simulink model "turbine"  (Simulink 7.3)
settings: Solver=ode23tb  StartTime=0.0  StopTime=1000  RelTol=1e-3
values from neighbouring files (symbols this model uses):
  c_d = 0.9658    [dynamic_main.m]    (also in Parameter.m = 1; Parameter_sim.m; static_main.m = inv(H3'*H3)*H3'*y3)
  d_Turb = 5.35    [dynamic_main.m]    (also in Parameter.m; Parameter_sim.m; static_main.m)
  I_IC = 0    [dynamic_main.m]    (also in Parameter.m; Parameter_sim.m; static_main.m)
  kappa = 8.7000e3    (= 8700)    [dynamic_main.m]    (also in Parameter.m = 1; Parameter_sim.m; static_main.m = inv(H4'*H4)*H4'*y4)
  L_net = 0.1    [dynamic_main.m]    (also in Parameter_sim.m; static_main.m)
  L_tot = L_net+L_G    (= 0.2)    [dynamic_main.m]    (also in Parameter.m; Parameter_sim.m)
  omega_IC = 0    [dynamic_main.m]    (also in Parameter.m; Parameter_sim.m; static_main.m)
  p_0 = 0    [dynamic_main.m]    (also in Parameter.m; Parameter_sim.m; static_main.m)
  R_net = 165    [dynamic_main.m]    (also in Parameter_sim.m; static_main.m)
  R_tot = R_net+R_G    (= 175)    [dynamic_main.m]    (also in Parameter.m; Parameter_sim.m)
  rho = 1000    [dynamic_main.m]    (also in Parameter.m; Parameter_sim.m; static_main.m)
  Theta = fminsearch(@(Theta)err_turbine(Theta,time_bb,p_F_bb,x_bb,omega_bb),Theta_0)    [dynamic_main.m]    (also in Parameter.m = 1; Parameter_sim.m = 5499.7)

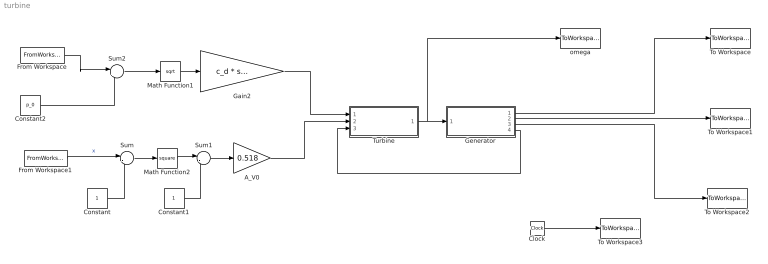
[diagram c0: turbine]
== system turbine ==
  A_V0 : Gain  Gain=0.518  ParameterDataType=sfix(16)  ParameterScaling=2^0  OutDataType=sfix(16)  OutScaling=2^0
  Clock : Clock
  Constant : Constant  OutDataType=sfix(16)  OutScaling=2^0
  Constant1 : Constant  OutDataType=sfix(16)  OutScaling=2^0
  Constant2 : Constant  Value=p_0  OutDataType=sfix(16)  OutScaling=2^0
  From Workspace : FromWorkspace  VariableName=[time_bb p_F_bb]  SampleTime=0
  From Workspace1 : FromWorkspace  VariableName=[time_bb x_bb]  SampleTime=0
  Gain2 : Gain  Gain=c_d * sqrt(2/rho)  ParameterDataType=sfix(16)  ParameterScaling=2^0  OutDataType=sfix(16)  OutScaling=2^0
  Generator : Subsystem
  Math Function1 : Math  Operator=sqrt  OutDataType=sfix(16)  OutScaling=2^0
  Math Function2 : Math  Operator=square  OutDataType=sfix(16)  OutScaling=2^0
  Sum : Sum  Inputs=|-+  OutDataType=sfix(16)  OutScaling=2^0
  Sum1 : Sum  Inputs=|-+  OutDataType=sfix(16)  OutScaling=2^0
  Sum2 : Sum  Inputs=|+-  OutDataType=sfix(16)  OutScaling=2^0
  To Workspace : ToWorkspace  VariableName=U  SampleTime=-1  SaveFormat=Array
  To Workspace1 : ToWorkspace  VariableName=I  SampleTime=-1  SaveFormat=Array
  To Workspace2 : ToWorkspace  VariableName=P  SampleTime=-1  SaveFormat=Array
  To Workspace3 : ToWorkspace  VariableName=time_sim  SampleTime=-1  SaveFormat=Array
  Turbine : Subsystem
  omega : ToWorkspace  VariableName=omega  SampleTime=-1  SaveFormat=Array
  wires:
  Turbine/1(omega) -> Generator/1(omega), omega/1
  Generator/1(U) -> To Workspace/1
  Generator/2(I) -> To Workspace1/1
  Generator/4(T_G) -> Turbine/3(T_G)
  Generator/3(P) -> To Workspace2/1
  Clock/1 -> To Workspace3/1
  Constant2/1 -> Sum2/2
  Sum2/1 -> Math Function1/1
  Math Function1/1 -> Gain2/1
  Gain2/1 -> Turbine/1(v_V)
  Constant/1 -> Sum/2
  Sum/1 -> Math Function2/1
  Constant1/1 -> Sum1/2
  Sum1/1 -> A_V0/1
  Math Function2/1 -> Sum1/1
  A_V0/1 -> Turbine/2(A_V)
  From Workspace1/1 -> Sum/1  "x"
  From Workspace/1 -> Sum2/1

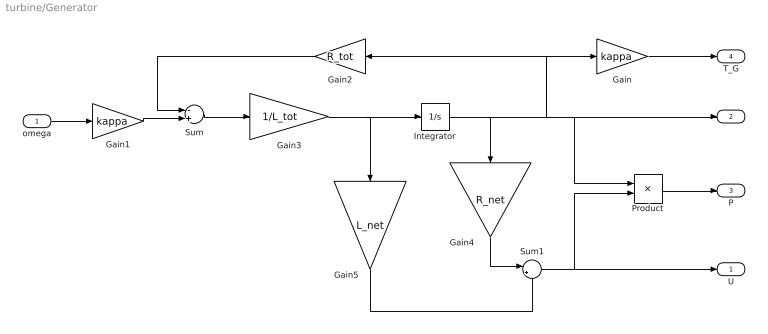
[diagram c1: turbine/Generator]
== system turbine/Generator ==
  omega : Inport  OutDataType=sfix(16)  OutScaling=2^0
  Gain : Gain  Gain=kappa  ParameterDataType=sfix(16)  ParameterScaling=2^0  OutDataType=sfix(16)  OutScaling=2^0
  Gain1 : Gain  Gain=kappa  ParameterDataType=sfix(16)  ParameterScaling=2^0  OutDataType=sfix(16)  OutScaling=2^0
  Gain2 : Gain  Gain=R_tot  ParameterDataType=sfix(16)  ParameterScaling=2^0  OutDataType=sfix(16)  OutScaling=2^0
  Gain3 : Gain  Gain=1/L_tot  ParameterDataType=sfix(16)  ParameterScaling=2^0  OutDataType=sfix(16)  OutScaling=2^0
  Gain4 : Gain  Gain=R_net  ParameterDataType=sfix(16)  ParameterScaling=2^0  OutDataType=sfix(16)  OutScaling=2^0
  Gain5 : Gain  Gain=L_net  ParameterDataType=sfix(16)  ParameterScaling=2^0  OutDataType=sfix(16)  OutScaling=2^0
  Integrator : Integrator  InitialCondition=I_IC
  Product : Product  OutDataType=sfix(16)  OutScaling=2^0
  Sum : Sum  Inputs=-+  OutDataType=sfix(16)  OutScaling=2^0
  Sum1 : Sum  Inputs=|++  OutDataType=sfix(16)  OutScaling=2^0
  U : Outport  OutDataType=sfix(16)  OutScaling=2^0
  I : Outport  Port=2  OutDataType=sfix(16)  OutScaling=2^0
  P : Outport  Port=3  OutDataType=sfix(16)  OutScaling=2^0
  T_G : Outport  Port=4  OutDataType=sfix(16)  OutScaling=2^0
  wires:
  Integrator/1 -> Gain/1, Gain2/1, I/1, Product/1, Gain4/1
  Gain/1 -> T_G/1
  omega/1 -> Gain1/1
  Gain2/1 -> Sum/1
  Gain1/1 -> Sum/2
  Sum/1 -> Gain3/1
  Gain3/1 -> Gain5/1, Integrator/1
  Sum1/1 -> U/1, Product/2
  Gain4/1 -> Sum1/1
  Gain5/1 -> Sum1/2
  Product/1 -> P/1

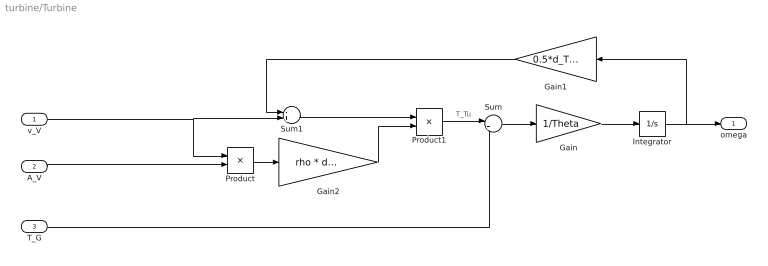
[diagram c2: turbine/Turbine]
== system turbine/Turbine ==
  v_V : Inport  OutDataType=sfix(16)  OutScaling=2^0
  A_V : Inport  Port=2  OutDataType=sfix(16)  OutScaling=2^0
  T_G : Inport  Port=3  OutDataType=sfix(16)  OutScaling=2^0
  Gain : Gain  Gain=1/Theta  ParameterDataType=sfix(16)  ParameterScaling=2^0  OutDataType=sfix(16)  OutScaling=2^0
  Gain1 : Gain  Gain=0.5*d_Turb  ParameterDataType=sfix(16)  ParameterScaling=2^0  OutDataType=sfix(16)  OutScaling=2^0
  Gain2 : Gain  Gain=rho * d_Turb  ParameterDataType=sfix(16)  ParameterScaling=2^0  OutDataType=sfix(16)  OutScaling=2^0
  Integrator : Integrator  InitialCondition=omega_IC
  Product : Product  OutDataType=sfix(16)  OutScaling=2^0
  Product1 : Product  OutDataType=sfix(16)  OutScaling=2^0
  Sum : Sum  Inputs=|+-  OutDataType=sfix(16)  OutScaling=2^0
  Sum1 : Sum  Inputs=-+  OutDataType=sfix(16)  OutScaling=2^0
  omega : Outport  OutDataType=sfix(16)  OutScaling=2^0
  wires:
  Integrator/1 -> omega/1, Gain1/1
  Gain/1 -> Integrator/1
  Sum/1 -> Gain/1
  T_G/1 -> Sum/2
  v_V/1 -> Product/1, Sum1/2
  A_V/1 -> Product/2
  Gain1/1 -> Sum1/1
  Product/1 -> Gain2/1
  Sum1/1 -> Product1/1
  Gain2/1 -> Product1/2
  Product1/1 -> Sum/1  "T_Tu"
